| IBIS file generated by GenIBIS.pl Version 3.24
|   j6plus
[IBIS ver]   5.0
[File name]   j6plus.ibs
[File Rev]   1.0.0
[Date]   Thu Jan 25, 2018, 13:15:8
[Source]   Data created at Texas Instruments
[Notes]   J6Plus ABZ IBIS Model Revision History
   Version 1.0.0, January 25th, 2018
   - Initial Release
   Note 1) Checked by IBISCHK5.
[Disclaimer] Please be aware that in the absence of a written agreement,
   Texas Instruments (TI) assumes no liability for: 1) the
   accuracy of the IBIS models provided to your company, 2) the
   proper functioning of these IBIS models in your design or for
   any resulting applications, or, 3) infringement of patents,
   copyrights, or intellectual property rights resulting from
   your use of these IBIS models. TI provides IBIS models as a
   service to our customers and therefore reserves the right to
   limit distribution of the IBIS models.
[Copyright]   Property of Texas Instruments Incorporated. Unauthorised
   reproduction and/or distribution is strictly prohibited. This
   product is protected under copyright law and trade secret law
   as an unpublished work. Created 2016,(C) Copyright 2016,
   Texas Instruments Incorporated., All Rights Reserved. These
   commodities are under the U.S. Government distribution license
   control.As such,they are not to be re-exported without the
   prior approval of the U.S. Department of Commerce.
|   Component j6plus
[Component]   j6plus
[Manufacturer]   Texas Instruments.
| Source IO level model revisions
|Model   Revision   Date
|DDR_SEIOPB_V   2.5   23 May 2014
|BC1833DV40DCPBFBHHVRXP1811_SSCEV   2.0   Sep 11, 2013
|BC1833DV40DCPBFBP1811_SSCEV   2.0   Sep 11, 2013
|BI2C1833DVFZP18_SSCEV   2.0   Sep 11, 2013
|BC1833DV40DCPBFBP1811_SSCEH   2.0   Sep 11, 2013
|DDR_DIFFIOPB_V   2.5   23 May 2014
|SATATX   1.0   Nov 07, 2012
|ACSPCIE_RX   0.5   May 16, 2012
|SDIO1833PB_H   1.0   Sep 21, 2011
|USB3_PCIEGEN1_PCIEGEN2_TX   1.0   Nov 07, 2012
|HDMITXPHY   0.8   Jul 12, 2011
|DDR_DIFFIOPB_H   2.5   23 May 2014
|IQ1833DVTCKPBFBP18LL_SSCEV   2.0   Sep 11, 2013
|BMLBLVDS18_SSCEH   1.0   Jun 13, 2013
|ILVDS18HY_SSCEH   1.0   Apr 04, 2013
|USB2PHYCORE_HMAV10GS80   0.8   July 13, 2011
|GANGARX   1   Sep 04, 2012
|IHHV1833DVHYP1811_SSCEV   1.0   Dec 24, 2012
|DDR_SEIOPB_H   2.5   23 May 2014
[Package]
|   typ   min   max
R_pkg   0.416310963675214   0.029876000000000000 0.885390000000000000
L_pkg   2.57707435897436E-009 0.000000000420200000 0.000000004843000000
C_pkg   1.29004209401709E-012 0.000000000000566900 0.000000000002000000
[Pin]   signal_name   model_name   R_pin   L_pin   C_pin
Y10   ATESTV   NC
G19   DCAN1_RX   Selector_1   0.122460000000000000 0.000000001020000000 0.000000000000844400
G20   DCAN1_TX   Selector_1   0.153960000000000000 0.000000001124000000 0.000000000000940000
Y18   DDR1_VREF0   NC
AC18   DDR1_CASN   Selector_15  0.164920000000000000 0.000000001265000000 0.000000000000943600
AF17   DDR1_BA0   Selector_15  0.301210000000000000 0.000000002001000000 0.000000000001255000
AF24   DDR1_D4   Selector_4   0.467920000000000000 0.000000002978000000 0.000000000001397000
AC27   DDR1_D20   Selector_4   0.577380000000000000 0.000000003559000000 0.000000000001579000
AC24   DDR1_D14   Selector_4   0.366310000000000000 0.000000002279000000 0.000000000001257000
AG25   DDR1_DQSN0   Selector_11  0.686690000000000000 0.000000003636000000 0.000000000001223000
AH25   DDR1_DQS0   Selector_9   0.686670000000000000 0.000000003663000000 0.000000000001216000
AG23   DDR1_A6   Selector_15  0.527210000000000000 0.000000003212000000 0.000000000001560000
AF18   DDR1_A13   Selector_15  0.350510000000000000 0.000000002185000000 0.000000000001282000
AF25   DDR1_D0   Selector_4   0.547110000000000000 0.000000003377000000 0.000000000001490000
Y23   DDR1_D26   Selector_4   0.272260000000000000 0.000000001860000000 0.000000000001192000
AE17   DDR1_A14   Selector_15  0.273350000000000000 0.000000001811000000 0.000000000001053000
AB18   DDR1_BA2   Selector_15  0.110020000000000000 0.000000000951200000 0.000000000000877200
AE28   DDR1_DQSN1   Selector_11  0.760100000000000000 0.000000003994000000 0.000000000001297000
Y22   DDR1_D25   Selector_4   0.243100000000000000 0.000000001796000000 0.000000000001094000
W23   DDR1_ECC_D3   Selector_4   0.310930000000000000 0.000000002177000000 0.000000000001181000
V24   DDR1_ECC_D5   Selector_4   0.304360000000000000 0.000000002061000000 0.000000000001069000
AE23   DDR1_D7   Selector_4   0.349920000000000000 0.000000002264000000 0.000000000001249000
Y26   DDR1_ECC_D7   Selector_4   0.475480000000000000 0.000000002872000000 0.000000000001589000
AF28   DDR1_D11   Selector_4   0.665540000000000000 0.000000003965000000 0.000000000001718000
AF27   DDR1_D9   Selector_4   0.600380000000000000 0.000000003672000000 0.000000000001622000
V25   DDR1_ECC_D6   Selector_4   0.398200000000000000 0.000000002464000000 0.000000000001225000
AB19   DDR1_A3   Selector_15  0.102890000000000000 0.000000000866100000 0.000000000000875200
AB23   DDR1_DQM1   Selector_24  0.300060000000000000 0.000000001913000000 0.000000000001147000
AA26   DDR1_D29   Selector_4   0.444900000000000000 0.000000002759000000 0.000000000001396000
AD21   DDR1_A10   Selector_15  0.232890000000000000 0.000000001597000000 0.000000000001048000
AC20   DDR1_A2   Selector_15  0.179280000000000000 0.000000001323000000 0.000000000001091000
AC19   DDR1_A1   Selector_15  0.195630000000000000 0.000000001384000000 0.000000000001014000
Y19   DDR1_D21   Selector_4   0.124200000000000000 0.000000001407000000 0.000000000000793300
AE21   DDR1_A7   Selector_15  0.276170000000000000 0.000000001894000000 0.000000000001188000
V20   DDR1_D16   Selector_4   0.029876000000000000 0.000000000420200000 0.000000000000566900
W20   DDR1_D17   Selector_4   0.140870000000000000 0.000000001414000000 0.000000000000882900
AC25   DDR1_D13   Selector_4   0.413520000000000000 0.000000002556000000 0.000000000001325000
AF20   DDR1_RASN   Selector_15  0.368020000000000000 0.000000002258000000 0.000000000001267000
AE20   DDR1_ODT0   Selector_15  0.355230000000000000 0.000000002143000000 0.000000000001225000
AC26   DDR1_DQM2   Selector_24  0.480350000000000000 0.000000002974000000 0.000000000001462000
AH21   DDR1_WEN   Selector_15  0.521940000000000000 0.000000003071000000 0.000000000001524000
AF26   DDR1_D1   Selector_4   0.528520000000000000 0.000000003223000000 0.000000000001524000
AA23   DDR1_D24   Selector_4   0.367330000000000000 0.000000002386000000 0.000000000001236000
AE18   DDR1_BA1   Selector_15  0.292490000000000000 0.000000001893000000 0.000000000001142000
AF21   DDR1_A4   Selector_15  0.411750000000000000 0.000000002543000000 0.000000000001330000
Y24   DDR1_D28   Selector_4   0.330980000000000000 0.000000002222000000 0.000000000001202000
AB28   DDR1_D18   Selector_4   0.589030000000000000 0.000000003678000000 0.000000000001605000
AG26   DDR1_D2   Selector_4   0.594910000000000000 0.000000003559000000 0.000000000001617000
AE26   DDR1_D12   Selector_4   0.534150000000000000 0.000000003309000000 0.000000000001512000
W19   DDR1_ECC_D2   Selector_4   0.121200000000000000 0.000000001451000000 0.000000000000911300
Y25   DDR1_ECC_D4   Selector_4   0.438840000000000000 0.000000002766000000 0.000000000001554000
AA24   DDR1_D27   Selector_4   0.365560000000000000 0.000000002344000000 0.000000000001341000
AD25   DDR1_D15   Selector_4   0.440700000000000000 0.000000002662000000 0.000000000001411000
AB27   DDR1_D22   Selector_4   0.526930000000000000 0.000000003352000000 0.000000000001471000
AD18   DDR1_A15   Selector_15  0.256150000000000000 0.000000001762000000 0.000000000001106000
V28   DDR1_DQSN_ECC   Selector_11  0.652950000000000000 0.000000003413000000 0.000000000001116000
AH24   DDR1_NCK   Selector_2   0.675840000000000000 0.000000003620000000 0.000000000001430000
AG21   DDR1_RST   Selector_15  0.485470000000000000 0.000000002873000000 0.000000000001461000
AH26   DDR1_D3   Selector_4   0.636390000000000000 0.000000003722000000 0.000000000001688000
AG27   DDR1_D10   Selector_4   0.660570000000000000 0.000000003855000000 0.000000000001682000
AH23   DDR1_CSN0   Selector_15  0.545150000000000000 0.000000003312000000 0.000000000001572000
V23   DDR1_ECC_D1   Selector_4   0.265250000000000000 0.000000001842000000 0.000000000000989700
AD27   DDR1_DQS2   Selector_9   0.736580000000000000 0.000000003833000000 0.000000000001273000
AD20   DDR1_A0   Selector_15  0.277790000000000000 0.000000001769000000 0.000000000001149000
AE22   DDR1_A9   Selector_15  0.329590000000000000 0.000000002164000000 0.000000000001191000
AC23   DDR1_D8   Selector_4   0.337500000000000000 0.000000002104000000 0.000000000001168000
AF22   DDR1_A8   Selector_15  0.388250000000000000 0.000000002470000000 0.000000000001364000
Y20   DDR1_D23   Selector_4   0.171330000000000000 0.000000001625000000 0.000000000000866800
AA25   DDR1_D30   Selector_4   0.444120000000000000 0.000000002721000000 0.000000000001354000
AE24   DDR1_D5   Selector_4   0.381750000000000000 0.000000002397000000 0.000000000001289000
AA28   DDR1_D31   Selector_4   0.570840000000000000 0.000000003446000000 0.000000000001566000
AD23   DDR1_DQM0   Selector_24  0.413750000000000000 0.000000002529000000 0.000000000001431000
Y28   DDR1_DQS3   Selector_9   0.680200000000000000 0.000000003597000000 0.000000000001212000
AD22   DDR1_A11   Selector_15  0.283590000000000000 0.000000001813000000 0.000000000001127000
W22   DDR1_ECC_D0   Selector_4   0.206760000000000000 0.000000001672000000 0.000000000001080000
AC28   DDR1_D19   Selector_4   0.610720000000000000 0.000000003757000000 0.000000000001645000
V26   DDR1_DQM_ECC   Selector_24  0.391490000000000000 0.000000002463000000 0.000000000001261000
AG24   DDR1_CK   Selector_23  0.669160000000000000 0.000000003598000000 0.000000000001402000
AG22   DDR1_CKE   Selector_15  0.492780000000000000 0.000000002955000000 0.000000000001478000
AE27   DDR1_DQS1   Selector_9   0.755390000000000000 0.000000003951000000 0.000000000001287000
AH22   DDR1_A5   Selector_15  0.522550000000000000 0.000000003169000000 0.000000000001523000
AF23   DDR1_D6   Selector_4   0.435010000000000000 0.000000002668000000 0.000000000001399000
AC21   DDR1_A12   Selector_15  0.134350000000000000 0.000000001044000000 0.000000000000979200
Y27   DDR1_DQSN3   Selector_11  0.684620000000000000 0.000000003563000000 0.000000000001218000
AA27   DDR1_DQM3   Selector_24  0.574580000000000000 0.000000003410000000 0.000000000001518000
AD28   DDR1_DQSN2   Selector_11  0.740220000000000000 0.000000003935000000 0.000000000001267000
V27   DDR1_DQS_ECC   Selector_9   0.648360000000000000 0.000000003393000000 0.000000000001064000
H23   DDR2_D8   Selector_4   0.240810000000000000 0.000000001716000000 0.000000000001047000
G27   DDR2_DQSN0   Selector_11  0.638590000000000000 0.000000003419000000 0.000000000001140000
H24   DDR2_D10   Selector_4   0.233120000000000000 0.000000001629000000 0.000000000000932500
E28   DDR2_D7   Selector_4   0.648570000000000000 0.000000004028000000 0.000000000001696000
T23   DDR2_RASN   Selector_24  0.211170000000000000 0.000000001627000000 0.000000000001110000
T28   DDR2_CK   Selector_19  0.650150000000000000 0.000000003469000000 0.000000000001406000
E26   DDR2_D0   Selector_4   0.521980000000000000 0.000000003242000000 0.000000000001414000
J23   DDR2_D21   Selector_4   0.190720000000000000 0.000000001472000000 0.000000000001064000
P24   DDR2_CSN0   Selector_24  0.246740000000000000 0.000000001653000000 0.000000000001115000
K27   DDR2_DQS2   Selector_9   0.568970000000000000 0.000000003027000000 0.000000000001107000
F24   DDR2_D3   Selector_4   0.244890000000000000 0.000000001861000000 0.000000000001070000
P25   DDR2_A6   Selector_24  0.312340000000000000 0.000000001986000000 0.000000000001205000
L27   DDR2_D24   Selector_4   0.449790000000000000 0.000000002892000000 0.000000000001395000
R24   DDR2_RST   Selector_24  0.241190000000000000 0.000000001815000000 0.000000000000818100
U27   DDR2_BA1   Selector_24  0.486910000000000000 0.000000003017000000 0.000000000001455000
L25   DDR2_D26   Selector_4   0.297020000000000000 0.000000002036000000 0.000000000001162000
H28   DDR2_DQSN1   Selector_11  0.612440000000000000 0.000000003233000000 0.000000000001147000
P22   DDR2_A5   Selector_24  0.108720000000000000 0.000000000951100000 0.000000000000841700
N20   DDR2_A7   Selector_24  0.087295000000000000 0.000000000837800000 0.000000000000973900
U28   DDR2_CASN   Selector_24  0.524570000000000000 0.000000003294000000 0.000000000001509000
R27   DDR2_A3   Selector_24  0.397600000000000000 0.000000002516000000 0.000000000001347000
R28   DDR2_A2   Selector_24  0.476310000000000000 0.000000002942000000 0.000000000001547000
N27   DDR2_A9   Selector_24  0.417770000000000000 0.000000002583000000 0.000000000001359000
J25   DDR2_D13   Selector_4   0.291620000000000000 0.000000001981000000 0.000000000001140000
T27   DDR2_NCK   Selector_6   0.645420000000000000 0.000000003416000000 0.000000000001404000
U22   DDR2_A15   Selector_24  0.216050000000000000 0.000000001636000000 0.000000000000993100
G25   DDR2_D1   Selector_4   0.309710000000000000 0.000000002121000000 0.000000000001364000
N22   DDR2_VREF0   NC
J20   DDR2_D23   Selector_4   0.124920000000000000 0.000000001332000000 0.000000000000792500
P26   DDR2_A11   Selector_24  0.383910000000000000 0.000000002413000000 0.000000000001405000
M26   DDR2_D31   Selector_4   0.362470000000000000 0.000000002349000000 0.000000000001268000
G28   DDR2_DQS0   Selector_9   0.636390000000000000 0.000000003436000000 0.000000000001162000
P27   DDR2_A8   Selector_24  0.441510000000000000 0.000000002655000000 0.000000000001401000
F26   DDR2_D4   Selector_4   0.407610000000000000 0.000000002693000000 0.000000000001340000
J24   DDR2_D15   Selector_4   0.231270000000000000 0.000000001586000000 0.000000000001063000
U26   DDR2_BA2   Selector_24  0.388360000000000000 0.000000002548000000 0.000000000001260000
K20   DDR2_D17   Selector_4   0.110100000000000000 0.000000000960400000 0.000000000000952900
K21   DDR2_D18   Selector_4   0.146240000000000000 0.000000001357000000 0.000000000000769300
F28   DDR2_DQM0   Selector_24  0.485980000000000000 0.000000003089000000 0.000000000001460000
F27   DDR2_D5   Selector_4   0.463800000000000000 0.000000003028000000 0.000000000001403000
H25   DDR2_D9   Selector_4   0.283610000000000000 0.000000001882000000 0.000000000001012000
E27   DDR2_D6   Selector_4   0.697810000000000000 0.000000004197000000 0.000000000001723000
N28   DDR2_A12   Selector_24  0.468070000000000000 0.000000002806000000 0.000000000001458000
M28   DDR2_DQS3   Selector_9   0.612940000000000000 0.000000003288000000 0.000000000001154000
R22   DDR2_A14   Selector_24  0.099049000000000000 0.000000000986200000 0.000000000000850000
F25   DDR2_D2   Selector_4   0.328350000000000000 0.000000002272000000 0.000000000001280000
R23   DDR2_ODT0   Selector_24  0.188980000000000000 0.000000001434000000 0.000000000000996600
U25   DDR2_WEN   Selector_24  0.329990000000000000 0.000000002165000000 0.000000000001199000
P23   DDR2_A4   Selector_24  0.186820000000000000 0.000000001421000000 0.000000000000995300
L22   DDR2_D16   Selector_4   0.160650000000000000 0.000000001265000000 0.000000000000862300
M25   DDR2_D30   Selector_4   0.310970000000000000 0.000000002031000000 0.000000000001158000
K28   DDR2_DQSN2   Selector_11  0.573880000000000000 0.000000003065000000 0.000000000001104000
T22   DDR2_A13   Selector_24  0.131960000000000000 0.000000001064000000 0.000000000000919200
L24   DDR2_D20   Selector_4   0.235900000000000000 0.000000001815000000 0.000000000001064000
U24   DDR2_CKE   Selector_24  0.387060000000000000 0.000000002414000000 0.000000000001258000
G26   DDR2_D12   Selector_4   0.412720000000000000 0.000000002652000000 0.000000000001301000
G24   DDR2_DQM1   Selector_24  0.324140000000000000 0.000000002183000000 0.000000000001192000
M24   DDR2_D29   Selector_4   0.238990000000000000 0.000000001702000000 0.000000000001075000
J26   DDR2_D14   Selector_4   0.365690000000000000 0.000000002376000000 0.000000000001274000
M27   DDR2_DQSN3   Selector_11  0.606620000000000000 0.000000003254000000 0.000000000001143000
L26   DDR2_D25   Selector_4   0.346940000000000000 0.000000002349000000 0.000000000001175000
N23   DDR2_A10   Selector_24  0.166950000000000000 0.000000001245000000 0.000000000001002000
M22   DDR2_DQM3   Selector_24  0.129140000000000000 0.000000001042000000 0.000000000000872100
R26   DDR2_A1   Selector_24  0.438110000000000000 0.000000002781000000 0.000000000001390000
H27   DDR2_DQS1   Selector_9   0.606290000000000000 0.000000003215000000 0.000000000001140000
H26   DDR2_D11   Selector_4   0.376180000000000000 0.000000002442000000 0.000000000001044000
K22   DDR2_D22   Selector_4   0.151900000000000000 0.000000001300000000 0.000000000000851000
M23   DDR2_D28   Selector_4   0.191100000000000000 0.000000001538000000 0.000000000000994800
R25   DDR2_A0   Selector_24  0.295990000000000000 0.000000001946000000 0.000000000001164000
K23   DDR2_DQM2   Selector_24  0.193660000000000000 0.000000001440000000 0.000000000000942300
L23   DDR2_D19   Selector_4   0.160130000000000000 0.000000001405000000 0.000000000000860500
U23   DDR2_BA0   Selector_24  0.217440000000000000 0.000000001679000000 0.000000000001004000
L28   DDR2_D27   Selector_4   0.467880000000000000 0.000000003012000000 0.000000000001388000
G21   EMU0   Selector_1   0.210670000000000000 0.000000001513000000 0.000000000001052000
D24   EMU1   Selector_1   0.610690000000000000 0.000000003477000000 0.000000000001687000
F20   GPIO6_15   Selector_1   0.217870000000000000 0.000000001581000000 0.000000000001032000
AB4   GPIO6_11   Selector_3   0.453040000000000000 0.000000002776000000 0.000000000001450000
E21   GPIO6_14   Selector_1   0.299290000000000000 0.000000001976000000 0.000000000001117000
AC5   GPIO6_10   Selector_3   0.515360000000000000 0.000000003043000000 0.000000000001473000
F21   GPIO6_16   Selector_1   0.266490000000000000 0.000000001815000000 0.000000000001092000
J4   GPMC_A24   Selector_3   0.291730000000000000 0.000000001896000000 0.000000000001168000
P1   GPMC_CS3   Selector_3   0.528930000000000000 0.000000003226000000 0.000000000001523000
M1   GPMC_AD3   Selector_3   0.477430000000000000 0.000000002985000000 0.000000000001442000
T2   GPMC_A14   Selector_3   0.492150000000000000 0.000000002952000000 0.000000000001463000
M7   GPMC_A20   Selector_3   0.156510000000000000 0.000000001381000000 0.000000000000860800
H2   GPMC_AD14   Selector_3   0.470220000000000000 0.000000002899000000 0.000000000001439000
J3   GPMC_AD13   Selector_3   0.360410000000000000 0.000000002239000000 0.000000000001258000
J1   GPMC_AD10   Selector_3   0.492680000000000000 0.000000002999000000 0.000000000001450000
J7   GPMC_A23   Selector_3   0.098787000000000000 0.000000000927100000 0.000000000000827700
P7   GPMC_CLK   Selector_3   0.121860000000000000 0.000000001057000000 0.000000000001006000
N6   GPMC_BEN0   Selector_3   0.206180000000000000 0.000000001474000000 0.000000000001071000
T6   GPMC_A2   Selector_3   0.308980000000000000 0.000000002202000000 0.000000000001105000
H5   GPMC_A27   Selector_3   0.251850000000000000 0.000000001711000000 0.000000000001110000
T1   GPMC_CS0   Selector_3   0.599210000000000000 0.000000003538000000 0.000000000001612000
T9   GPMC_A1   Selector_3   0.343020000000000000 0.000000002821000000 0.000000000001436000
M4   GPMC_BEN1   Selector_3   0.300700000000000000 0.000000001986000000 0.000000000001158000
H4   GPMC_A26   Selector_3   0.296060000000000000 0.000000001958000000 0.000000000001176000
L1   GPMC_AD8   Selector_3   0.492080000000000000 0.000000003001000000 0.000000000001454000
R9   GPMC_A5   Selector_3   0.197610000000000000 0.000000001861000000 0.000000000000991500
J5   GPMC_A21   Selector_3   0.237000000000000000 0.000000001696000000 0.000000000001036000
M3   GPMC_WEN   Selector_3   0.371310000000000000 0.000000002441000000 0.000000000001276000
K7   GPMC_A19   Selector_3   0.111770000000000000 0.000000001116000000 0.000000000000855500
P3   GPMC_A17   Selector_3   0.402580000000000000 0.000000002572000000 0.000000000001333000
K2   GPMC_AD9   Selector_3   0.395330000000000000 0.000000002415000000 0.000000000001328000
L5   GPMC_AD2   Selector_3   0.263700000000000000 0.000000001806000000 0.000000000001092000
R4   GPMC_A9   Selector_3   0.384180000000000000 0.000000002422000000 0.000000000001310000
H3   GPMC_AD15   Selector_3   0.403470000000000000 0.000000002535000000 0.000000000001326000
M5   GPMC_OEN_REN   Selector_3   0.234930000000000000 0.000000001637000000 0.000000000001073000
M6   GPMC_AD0   Selector_3   0.260090000000000000 0.000000001821000000 0.000000000001146000
R6   GPMC_A0   Selector_3   0.288940000000000000 0.000000001989000000 0.000000000001085000
M2   GPMC_AD1   Selector_3   0.412900000000000000 0.000000002609000000 0.000000000001347000
T7   GPMC_A3   Selector_3   0.241280000000000000 0.000000001799000000 0.000000000001191000
N2   GPMC_WAIT0   Selector_3   0.427140000000000000 0.000000002701000000 0.000000000001366000
P6   GPMC_A4   Selector_3   0.194950000000000000 0.000000001458000000 0.000000000000890200
K6   GPMC_A22   Selector_3   0.205000000000000000 0.000000001568000000 0.000000000001025000
R5   GPMC_A6   Selector_3   0.339370000000000000 0.000000002271000000 0.000000000001307000
L4   GPMC_AD5   Selector_3   0.275690000000000000 0.000000001812000000 0.000000000001154000
P2   GPMC_CS2   Selector_3   0.439120000000000000 0.000000002752000000 0.000000000001408000
J2   GPMC_AD11   Selector_3   0.412050000000000000 0.000000002557000000 0.000000000001335000
L6   GPMC_AD4   Selector_3   0.268580000000000000 0.000000001799000000 0.000000000001168000
N1   GPMC_ADVN_ALE   Selector_3   0.517060000000000000 0.000000003232000000 0.000000000001496000
P5   GPMC_A7   Selector_3   0.276060000000000000 0.000000001849000000 0.000000000000872300
J6   GPMC_A25   Selector_3   0.191900000000000000 0.000000001431000000 0.000000000000966200
L2   GPMC_AD7   Selector_3   0.401480000000000000 0.000000002515000000 0.000000000001340000
L3   GPMC_AD6   Selector_3   0.358640000000000000 0.000000002324000000 0.000000000001271000
H6   GPMC_CS1   Selector_3   0.168370000000000000 0.000000001280000000 0.000000000000964700
R3   GPMC_A13   Selector_3   0.426150000000000000 0.000000002676000000 0.000000000001378000
U2   GPMC_A15   Selector_3   0.577050000000000000 0.000000003437000000 0.000000000001609000
U1   GPMC_A16   Selector_3   0.588670000000000000 0.000000003468000000 0.000000000001629000
N9   GPMC_A10   Selector_3   0.167700000000000000 0.000000001421000000 0.000000000000893300
R2   GPMC_A18   Selector_3   0.477360000000000000 0.000000002858000000 0.000000000001460000
P4   GPMC_A12   Selector_3   0.317910000000000000 0.000000002057000000 0.000000000001226000
N7   GPMC_A8   Selector_3   0.176810000000000000 0.000000001368000000 0.000000000000797400
P9   GPMC_A11   Selector_3   0.154040000000000000 0.000000001316000000 0.000000000000863000
H1   GPMC_AD12   Selector_3   0.619770000000000000 0.000000003715000000 0.000000000001581000
AH16   HDMI1_CLOCKY   ibis_tmdsm_M#44   0.571920000000000000 0.000000003071000000 0.000000000001110000
AH19   HDMI1_DATA2Y   ibis_tmdsm_M#44   0.649690000000000000 0.000000003339000000 0.000000000001189000
AH17   HDMI1_DATA0Y   ibis_tmdsm_M#44   0.568420000000000000 0.000000003074000000 0.000000000001104000
AH18   HDMI1_DATA1Y   ibis_tmdsm_M#44   0.613430000000000000 0.000000003241000000 0.000000000001156000
AG18   HDMI1_DATA1X   ibis_tmdsp_M#43   0.607690000000000000 0.000000003192000000 0.000000000001158000
AG17   HDMI1_DATA0X   ibis_tmdsp_M#43   0.557830000000000000 0.000000003023000000 0.000000000001077000
AG16   HDMI1_CLOCKX   ibis_tmdsp_M#43   0.561720000000000000 0.000000003002000000 0.000000000001066000
AG19   HDMI1_DATA2X   ibis_tmdsp_M#43   0.646780000000000000 0.000000003295000000 0.000000000001187000
C20   I2C1_SCL   Selector_21  0.392320000000000000 0.000000002451000000 0.000000000001342000
C25   I2C2_SDA   Selector_21  0.683350000000000000 0.000000003941000000 0.000000000001770000
F17   I2C2_SCL   Selector_21  0.175220000000000000 0.000000001289000000 0.000000000001037000
C21   I2C1_SDA   Selector_21  0.429010000000000000 0.000000002605000000 0.000000000001399000
AG15   LJCB_CLKP   ACSPCIE_RX_M#753   0.558230000000000000 0.000000003040000000 0.000000000001286000
AH15   LJCB_CLKN   ACSPCIE_RX_M#753   0.576810000000000000 0.000000003218000000 0.000000000001301000
F14   MCASP1_AXR15   Selector_1   0.190290000000000000 0.000000001469000000 0.000000000000967800
J14   MCASP1_FSR   Selector_1   0.086283000000000000 0.000000000988700000 0.000000000000881600
A12   MCASP1_AXR11   Selector_1   0.509860000000000000 0.000000003239000000 0.000000000001463000
G12   MCASP1_AXR0   Selector_1   0.096733000000000000 0.000000000857600000 0.000000000000847800
B12   MCASP1_AXR8   Selector_1   0.402560000000000000 0.000000002602000000 0.000000000001334000
A11   MCASP1_AXR9   Selector_1   0.518700000000000000 0.000000003316000000 0.000000000001489000
C12   MCASP1_AXR6   Selector_1   0.355690000000000000 0.000000002295000000 0.000000000001244000
G13   MCASP1_AXR2   Selector_1   0.076957000000000000 0.000000000819900000 0.000000000000812800
A13   MCASP1_AXR13   Selector_1   0.480130000000000000 0.000000003007000000 0.000000000001427000
G14   MCASP1_AXR14   Selector_1   0.077843000000000000 0.000000000814500000 0.000000000000771000
F13   MCASP1_AXR5   Selector_1   0.170500000000000000 0.000000001298000000 0.000000000000921700
C14   MCASP1_ACLKX   Selector_1   0.346490000000000000 0.000000002246000000 0.000000000001229000
D12   MCASP1_AXR7   Selector_1   0.320340000000000000 0.000000002092000000 0.000000000001152000
B13   MCASP1_AXR10   Selector_1   0.386000000000000000 0.000000002502000000 0.000000000001276000
E14   MCASP1_AXR12   Selector_1   0.218290000000000000 0.000000001518000000 0.000000000001036000
F12   MCASP1_AXR1   Selector_1   0.186440000000000000 0.000000001508000000 0.000000000000984500
E12   MCASP1_AXR4   Selector_1   0.219410000000000000 0.000000001479000000 0.000000000001057000
D14   MCASP1_FSX   Selector_1   0.260650000000000000 0.000000001753000000 0.000000000001137000
J11   MCASP1_AXR3   Selector_1   0.150440000000000000 0.000000001402000000 0.000000000001091000
B14   MCASP1_ACLKR   Selector_1   0.380010000000000000 0.000000002357000000 0.000000000001292000
A20   MCASP2_FSR   Selector_1   0.708330000000000000 0.000000004296000000 0.000000000001766000
E15   MCASP2_ACLKR   Selector_1   0.201150000000000000 0.000000001406000000 0.000000000001029000
C15   MCASP2_AXR2   Selector_1   0.342120000000000000 0.000000002164000000 0.000000000001222000
A19   MCASP2_ACLKX   Selector_1   0.566880000000000000 0.000000003498000000 0.000000000001593000
A17   MCASP2_AXR7   Selector_1   0.553650000000000000 0.000000003422000000 0.000000000001572000
B15   MCASP2_AXR0   Selector_1   0.385200000000000000 0.000000002385000000 0.000000000001313000
B17   MCASP2_AXR6   Selector_1   0.470300000000000000 0.000000002989000000 0.000000000001432000
B16   MCASP2_AXR5   Selector_1   0.458270000000000000 0.000000002833000000 0.000000000001400000
A16   MCASP2_AXR3   Selector_1   0.507840000000000000 0.000000003115000000 0.000000000001494000
D15   MCASP2_AXR4   Selector_1   0.281870000000000000 0.000000001718000000 0.000000000001139000
A18   MCASP2_FSX   Selector_1   0.589690000000000000 0.000000003622000000 0.000000000001596000
A15   MCASP2_AXR1   Selector_1   0.479020000000000000 0.000000002865000000 0.000000000001472000
C17   MCASP3_AXR1   Selector_1   0.359750000000000000 0.000000002305000000 0.000000000001310000
F15   MCASP3_FSX   Selector_1   0.210910000000000000 0.000000001494000000 0.000000000001057000
B18   MCASP3_ACLKX   Selector_1   0.457210000000000000 0.000000002865000000 0.000000000001458000
B19   MCASP3_AXR0   Selector_1   0.514140000000000000 0.000000003138000000 0.000000000001497000
A21   MCASP4_FSX   Selector_1   0.611460000000000000 0.000000003634000000 0.000000000001675000
C18   MCASP4_ACLKX   Selector_1   0.493680000000000000 0.000000002970000000 0.000000000001441000
D17   MCASP4_AXR1   Selector_1   0.325750000000000000 0.000000002066000000 0.000000000001225000
G16   MCASP4_AXR0   Selector_1   0.076727000000000000 0.000000000726000000 0.000000000000842000
AB9   MCASP5_FSX   Selector_3   0.427290000000000000 0.000000003018000000 0.000000000001279000
AB3   MCASP5_AXR0   Selector_3   0.525870000000000000 0.000000003124000000 0.000000000001554000
AA3   MCASP5_ACLKX   Selector_3   0.470920000000000000 0.000000002967000000 0.000000000001422000
AA4   MCASP5_AXR1   Selector_3   0.414350000000000000 0.000000002573000000 0.000000000001374000
V1   MDIO_MCLK   Selector_3   0.575280000000000000 0.000000003382000000 0.000000000001595000
U4   MDIO_D   Selector_3   0.363390000000000000 0.000000002348000000 0.000000000001358000
AA1   MLBP_DAT_P   Selector_8   0.781090000000000000 0.000000004160000000 0.000000000001226000
AC1   MLBP_SIG_P   Selector_8   0.885390000000000000 0.000000004408000000 0.000000000001421000
AB2   MLBP_CLK_N   Selector_17  0.835580000000000000 0.000000004318000000 0.000000000001591000
AC2   MLBP_SIG_N   Selector_8   0.879920000000000000 0.000000004425000000 0.000000000001432000
AB1   MLBP_CLK_P   Selector_17  0.842990000000000000 0.000000004299000000 0.000000000001596000
AA2   MLBP_DAT_N   Selector_8   0.773220000000000000 0.000000004134000000 0.000000000001228000
Y9   MMC1_SDWP   Selector_3   0.191560000000000000 0.000000001936000000 0.000000000001015000
AA5   MMC1_DAT2   Selector_10  0.420790000000000000 0.000000002707000000 0.000000000001413000
W7   MMC1_SDCD   Selector_3   0.246510000000000000 0.000000001530000000 0.000000000000995200
W6   MMC1_CLK   Selector_10  0.283310000000000000 0.000000001911000000 0.000000000001270000
Y3   MMC1_DAT3   Selector_10  0.451260000000000000 0.000000002587000000 0.000000000001476000
Y4   MMC1_DAT1   Selector_10  0.378740000000000000 0.000000002378000000 0.000000000001391000
Y6   MMC1_CMD   Selector_10  0.355210000000000000 0.000000002326000000 0.000000000001405000
AA6   MMC1_DAT0   Selector_10  0.445360000000000000 0.000000002962000000 0.000000000001431000
AC6   MMC3_DAT1   Selector_3   0.462550000000000000 0.000000002769000000 0.000000000001117000
AC8   MMC3_DAT4   Selector_3   0.501240000000000000 0.000000003198000000 0.000000000001483000
AC3   MMC3_DAT3   Selector_3   0.559820000000000000 0.000000003309000000 0.000000000001605000
AB5   MMC3_DAT7   Selector_3   0.399900000000000000 0.000000002478000000 0.000000000001330000
AC7   MMC3_DAT0   Selector_3   0.405150000000000000 0.000000002579000000 0.000000000001270000
AD6   MMC3_DAT5   Selector_3   0.499280000000000000 0.000000002984000000 0.000000000001556000
AC4   MMC3_CMD   Selector_3   0.528400000000000000 0.000000003167000000 0.000000000001530000
AC9   MMC3_DAT2   Selector_3   0.471100000000000000 0.000000003188000000 0.000000000001446000
AB8   MMC3_DAT6   Selector_3   0.396960000000000000 0.000000002795000000 0.000000000001086000
AD4   MMC3_CLK   Selector_3   0.538290000000000000 0.000000003176000000 0.000000000001549000
D21   NMIN   Selector_20  0.365900000000000000 0.000000002288000000 0.000000000001287000
Y11   ON_OFF   Selector_16  0.179250000000000000 0.000000001754000000 0.000000000000818900
AG13   PCIE_RXN0   usb3rx_M#227   0.531380000000000000 0.000000002953000000 0.000000000001044000
AG14   PCIE_TXN0   Selector_22  0.556410000000000000 0.000000003016000000 0.000000000001102000
AG12   PCIE_TXN1   Selector_22  0.518000000000000000 0.000000002903000000 0.000000000001015000
AH12   PCIE_TXP1   Selector_7   0.530450000000000000 0.000000002963000000 0.000000000001058000
AH14   PCIE_TXP0   Selector_7   0.569920000000000000 0.000000003126000000 0.000000000001098000
AG11   PCIE_RXN1   usb3rx_M#227   0.558570000000000000 0.000000003010000000 0.000000000001092000
AH13   PCIE_RXP0   usb3rx_M#227   0.542350000000000000 0.000000003012000000 0.000000000001069000
AH11   PCIE_RXP1   usb3rx_M#227   0.563190000000000000 0.000000003075000000 0.000000000001090000
F22   PORZ   Selector_14  0.354010000000000000 0.000000002167000000 0.000000000001286000
E23   RESETN   Selector_20  0.460550000000000000 0.000000002729000000 0.000000000001422000
W9   RGMII0_TXC   Selector_3   0.258630000000000000 0.000000002697000000 0.000000000001209000
V3   RGMII0_RXD2   Selector_3   0.458120000000000000 0.000000002759000000 0.000000000001455000
V6   RGMII0_TXD1   Selector_3   0.283890000000000000 0.000000002098000000 0.000000000001213000
V4   RGMII0_RXD3   Selector_3   0.367210000000000000 0.000000002569000000 0.000000000001400000
U5   RGMII0_RXC   Selector_3   0.301060000000000000 0.000000002086000000 0.000000000001273000
V5   RGMII0_RXCTL   Selector_3   0.306540000000000000 0.000000002144000000 0.000000000001199000
U7   RGMII0_TXD2   Selector_3   0.183830000000000000 0.000000001727000000 0.000000000000992500
U6   RGMII0_TXD0   Selector_3   0.255220000000000000 0.000000001952000000 0.000000000001044000
V9   RGMII0_TXCTL   Selector_3   0.211760000000000000 0.000000002050000000 0.000000000001075000
V7   RGMII0_TXD3   Selector_3   0.265520000000000000 0.000000002023000000 0.000000000001220000
W2   RGMII0_RXD0   Selector_3   0.565410000000000000 0.000000003231000000 0.000000000001613000
Y2   RGMII0_RXD1   Selector_3   0.604960000000000000 0.000000003536000000 0.000000000001663000
U3   RMII_MHZ_50_CLK   Selector_3   0.436800000000000000 0.000000002686000000 0.000000000001388000
F23   RSTOUTN   Selector_5   0.441700000000000000 0.000000002586000000 0.000000000001410000
AD14   RTC_OSC_XO   NC
AF14   RTC_ISO   Selector_14  0.336170000000000000 0.000000002277000000 0.000000000001204000
AB17   RTC_PORZ   Selector_14  0.129750000000000000 0.000000001225000000 0.000000000000787600
AE14   RTC_OSC_XI_CLKIN32   NC
E18   RTCK   Selector_5   0.224230000000000000 0.000000001557000000 0.000000000001079000
AG9   SATA1_RXP0   usb3rx_M#227   0.604150000000000000 0.000000003183000000 0.000000000001105000
AH10   SATA1_TXP0   sata_tx_M#752   0.576430000000000000 0.000000003093000000 0.000000000001105000
AH9   SATA1_RXN0   usb3rx_M#227   0.605090000000000000 0.000000003165000000 0.000000000001136000
AG10   SATA1_TXN0   sata_tx_M#752   0.567160000000000000 0.000000003086000000 0.000000000001069000
B20   SPI1_CS3   Selector_1   0.496050000000000000 0.000000002978000000 0.000000000001515000
A25   SPI1_SCLK   Selector_1   0.787960000000000000 0.000000004556000000 0.000000000001948000
F16   SPI1_D1   Selector_1   0.142940000000000000 0.000000001120000000 0.000000000000989800
A24   SPI1_CS0   Selector_1   0.769980000000000000 0.000000004267000000 0.000000000001919000
B21   SPI1_CS2   Selector_1   0.528490000000000000 0.000000003101000000 0.000000000001554000
A22   SPI1_CS1   Selector_1   0.652610000000000000 0.000000003696000000 0.000000000001733000
B25   SPI1_D0   Selector_1   0.810960000000000000 0.000000004560000000 0.000000000001990000
A26   SPI2_SCLK   Selector_1   0.849820000000000000 0.000000004843000000 0.000000000001993000
B22   SPI2_D1   Selector_1   0.584400000000000000 0.000000003383000000 0.000000000001634000
B24   SPI2_CS0   Selector_1   0.701580000000000000 0.000000003903000000 0.000000000001840000
G17   SPI2_D0   Selector_1   0.056831000000000000 0.000000000712400000 0.000000000000827500
E20   TCLK   Selector_12  0.295540000000000000 0.000000001906000000 0.000000000001138000
D23   TDI   Selector_20  0.527150000000000000 0.000000003065000000 0.000000000001540000
F19   TDO   Selector_5   0.196280000000000000 0.000000001345000000 0.000000000000994000
F18   TMS   Selector_20  0.190300000000000000 0.000000001326000000 0.000000000000976600
D20   TRSTN   Selector_20  0.322270000000000000 0.000000001987000000 0.000000000001184000
B27   UART1_RXD   Selector_1   0.686360000000000000 0.000000003917000000 0.000000000001721000
E25   UART1_CTSN   Selector_1   0.486850000000000000 0.000000002961000000 0.000000000001425000
C27   UART1_RTSN   Selector_1   0.651470000000000000 0.000000003794000000 0.000000000001703000
C26   UART1_TXD   Selector_1   0.608100000000000000 0.000000003623000000 0.000000000001603000
D27   UART2_CTSN   Selector_1   0.592850000000000000 0.000000003685000000 0.000000000001582000
D28   UART2_RXD   Selector_1   0.656850000000000000 0.000000004017000000 0.000000000001678000
D26   UART2_TXD   Selector_1   0.551860000000000000 0.000000003356000000 0.000000000001546000
C28   UART2_RTSN   Selector_1   0.703820000000000000 0.000000004178000000 0.000000000001726000
Y1   UART3_TXD   Selector_3   0.654740000000000000 0.000000003698000000 0.000000000001703000
V2   UART3_RXD   Selector_3   0.531070000000000000 0.000000003145000000 0.000000000001531000
AF12   USB_RXN0   usb3rx_M#227   0.355930000000000000 0.000000002364000000 0.000000000001064000
AD11   USB_TXP0   Selector_7   0.262330000000000000 0.000000001701000000 0.000000000000872400
AE12   USB_RXP0   usb3rx_M#227   0.348500000000000000 0.000000002272000000 0.000000000001044000
AC11   USB_TXN0   Selector_22  0.264110000000000000 0.000000001718000000 0.000000000000859300
AB10   USB1_DRVVBUS   Selector_3   0.222820000000000000 0.000000001650000000 0.000000000000936900
AD12   USB1_DP   Selector_13  0.245510000000000000 0.000000001902000000 0.000000000001012000
AC12   USB1_DM   Selector_18  0.230880000000000000 0.000000001907000000 0.000000000001013000
AE11   USB2_DP   Selector_13  0.406130000000000000 0.000000002386000000 0.000000000001033000
AF11   USB2_DM   Selector_18  0.414690000000000000 0.000000002457000000 0.000000000001031000
AC10   USB2_DRVVBUS   Selector_3   0.232040000000000000 0.000000001753000000 0.000000000000961100
AG4   VIN1A_D8   Selector_3   0.644140000000000000 0.000000003768000000 0.000000000001745000
AG8   VIN1A_CLK0   Selector_3   0.456950000000000000 0.000000002811000000 0.000000000001382000
AE2   VIN1A_D20   Selector_3   0.705280000000000000 0.000000004135000000 0.000000000001794000
AE9   VIN1A_HSYNC0   Selector_3   0.343420000000000000 0.000000002201000000 0.000000000001284000
AF3   VIN1A_D14   Selector_3   0.709310000000000000 0.000000004142000000 0.000000000001772000
AG5   VIN1A_D11   Selector_3   0.612550000000000000 0.000000003636000000 0.000000000001668000
AE5   VIN1A_D18   Selector_3   0.541150000000000000 0.000000003229000000 0.000000000001581000
AH3   VIN1A_D4   Selector_3   0.723470000000000000 0.000000004088000000 0.000000000001860000
AH7   VIN1B_CLK1   Selector_3   0.518630000000000000 0.000000003116000000 0.000000000001473000
AG3   VIN1A_D10   Selector_3   0.722080000000000000 0.000000004143000000 0.000000000001848000
AF6   VIN1A_D13   Selector_3   0.557040000000000000 0.000000003335000000 0.000000000001558000
AF2   VIN1A_D12   Selector_3   0.739150000000000000 0.000000004170000000 0.000000000001899000
AE3   VIN1A_D17   Selector_3   0.610430000000000000 0.000000003619000000 0.000000000001679000
AG6   VIN1A_D6   Selector_3   0.560780000000000000 0.000000003377000000 0.000000000001594000
AH4   VIN1A_D7   Selector_3   0.685090000000000000 0.000000004037000000 0.000000000001791000
AF8   VIN1A_VSYNC0   Selector_3   0.433520000000000000 0.000000002615000000 0.000000000001417000
AF4   VIN1A_D15   Selector_3   0.614510000000000000 0.000000003576000000 0.000000000001665000
AE1   VIN1A_D19   Selector_3   0.733440000000000000 0.000000004273000000 0.000000000001879000
AE6   VIN1A_D21   Selector_3   0.511380000000000000 0.000000003177000000 0.000000000001483000
AD3   VIN1A_D23   Selector_3   0.623830000000000000 0.000000003860000000 0.000000000001639000
AD8   VIN1A_D1   Selector_3   0.290910000000000000 0.000000001865000000 0.000000000001133000
AF1   VIN1A_D16   Selector_3   0.818720000000000000 0.000000004565000000 0.000000000002000000
AG7   VIN1A_D2   Selector_3   0.501510000000000000 0.000000002956000000 0.000000000001484000
AF9   VIN1A_FLD0   Selector_3   0.425880000000000000 0.000000002833000000 0.000000000001425000
AG2   VIN1A_D9   Selector_3   0.762120000000000000 0.000000004188000000 0.000000000001921000
AH5   VIN1A_D5   Selector_3   0.623950000000000000 0.000000003706000000 0.000000000001726000
AH6   VIN1A_D3   Selector_3   0.600380000000000000 0.000000003620000000 0.000000000001657000
AE8   VIN1A_D0   Selector_3   0.390070000000000000 0.000000002410000000 0.000000000001280000
AD2   VIN1A_D22   Selector_3   0.654400000000000000 0.000000003917000000 0.000000000001660000
AD9   VIN1A_DE0   Selector_3   0.268050000000000000 0.000000001969000000 0.000000000001134000
C4   VIN2A_D15   Selector_1   0.511230000000000000 0.000000003069000000 0.000000000001533000
C5   VIN2A_D18   Selector_1   0.480720000000000000 0.000000002882000000 0.000000000001486000
B3   VIN2A_D20   Selector_1   0.642120000000000000 0.000000003706000000 0.000000000001600000
F6   VIN2A_D11   Selector_1   0.316620000000000000 0.000000002010000000 0.000000000001196000
F3   VIN2A_D1   Selector_1   0.444350000000000000 0.000000002731000000 0.000000000001385000
E4   VIN2A_D7   Selector_1   0.418800000000000000 0.000000002532000000 0.000000000001369000
B2   VIN2A_D16   Selector_1   0.673200000000000000 0.000000003755000000 0.000000000001756000
A4   VIN2A_D23   Selector_1   0.631730000000000000 0.000000003677000000 0.000000000001681000
E1   VIN2A_CLK0   Selector_1   0.551850000000000000 0.000000003191000000 0.000000000001568000
D3   VIN2A_D10   Selector_1   0.531630000000000000 0.000000003156000000 0.000000000001548000
C3   VIN2A_D14   Selector_1   0.553320000000000000 0.000000003274000000 0.000000000001586000
D2   VIN2A_D4   Selector_1   0.546620000000000000 0.000000003238000000 0.000000000001578000
C1   VIN2A_D6   Selector_1   0.660820000000000000 0.000000003779000000 0.000000000001730000
G2   VIN2A_DE0   Selector_1   0.440660000000000000 0.000000002654000000 0.000000000001401000
F2   VIN2A_D0   Selector_1   0.481100000000000000 0.000000002842000000 0.000000000001430000
E6   VIN2A_D9   Selector_1   0.319700000000000000 0.000000001995000000 0.000000000001193000
C2   VIN2A_D13   Selector_1   0.612930000000000000 0.000000003553000000 0.000000000001570000
B4   VIN2A_D21   Selector_1   0.594510000000000000 0.000000003528000000 0.000000000001637000
E2   VIN2A_D3   Selector_1   0.521090000000000000 0.000000003053000000 0.000000000001528000
A3   VIN2A_D19   Selector_1   0.706960000000000000 0.000000003981000000 0.000000000001836000
D6   VIN2A_D17   Selector_1   0.378640000000000000 0.000000002353000000 0.000000000001312000
D1   VIN2A_D2   Selector_1   0.594670000000000000 0.000000003478000000 0.000000000001643000
D5   VIN2A_D12   Selector_1   0.399700000000000000 0.000000002471000000 0.000000000001323000
F5   VIN2A_D8   Selector_1   0.343010000000000000 0.000000002144000000 0.000000000001260000
B5   VIN2A_D22   Selector_1   0.526690000000000000 0.000000003082000000 0.000000000001533000
G6   VIN2A_VSYNC0   Selector_1   0.209530000000000000 0.000000001429000000 0.000000000001050000
G1   VIN2A_HSYNC0   Selector_1   0.493400000000000000 0.000000002895000000 0.000000000001474000
H7   VIN2A_FLD0   Selector_1   0.106300000000000000 0.000000000881100000 0.000000000000856300
F4   VIN2A_D5   Selector_1   0.391250000000000000 0.000000002425000000 0.000000000001329000
A8   VOUT1_D19   Selector_1   0.530670000000000000 0.000000003221000000 0.000000000001549000
E7   VOUT1_D7   Selector_1   0.383540000000000000 0.000000002382000000 0.000000000001351000
B8   VOUT1_D17   Selector_1   0.463940000000000000 0.000000002853000000 0.000000000001450000
B11   VOUT1_FLD   Selector_1   0.419930000000000000 0.000000002678000000 0.000000000001364000
C9   VOUT1_D20   Selector_1   0.415950000000000000 0.000000002694000000 0.000000000001327000
D9   VOUT1_D9   Selector_1   0.314710000000000000 0.000000002033000000 0.000000000001184000
C6   VOUT1_D13   Selector_1   0.538220000000000000 0.000000003168000000 0.000000000001528000
F10   VOUT1_D2   Selector_1   0.148300000000000000 0.000000001140000000 0.000000000000954900
F8   VOUT1_D6   Selector_1   0.362190000000000000 0.000000002239000000 0.000000000001301000
G11   VOUT1_D3   Selector_1   0.102570000000000000 0.000000000940500000 0.000000000000854500
B10   VOUT1_DE   Selector_1   0.457370000000000000 0.000000002943000000 0.000000000001364000
A5   VOUT1_D12   Selector_1   0.661750000000000000 0.000000003757000000 0.000000000001739000
F9   VOUT1_D5   Selector_1   0.307330000000000000 0.000000001950000000 0.000000000001215000
A9   VOUT1_D21   Selector_1   0.512710000000000000 0.000000003171000000 0.000000000001506000
E11   VOUT1_VSYNC   Selector_1   0.276370000000000000 0.000000001878000000 0.000000000001135000
B9   VOUT1_D22   Selector_1   0.470440000000000000 0.000000003015000000 0.000000000001393000
E8   VOUT1_D8   Selector_1   0.353540000000000000 0.000000002239000000 0.000000000001273000
E9   VOUT1_D4   Selector_1   0.254110000000000000 0.000000001732000000 0.000000000001108000
D7   VOUT1_D10   Selector_1   0.454260000000000000 0.000000002778000000 0.000000000001428000
C11   VOUT1_HSYNC   Selector_1   0.389250000000000000 0.000000002573000000 0.000000000001265000
A7   VOUT1_D18   Selector_1   0.575250000000000000 0.000000003342000000 0.000000000001617000
C7   VOUT1_D15   Selector_1   0.497340000000000000 0.000000002985000000 0.000000000001513000
F11   VOUT1_D0   Selector_1   0.115820000000000000 0.000000001074000000 0.000000000000945700
A10   VOUT1_D23   Selector_1   0.494740000000000000 0.000000003097000000 0.000000000001475000
C8   VOUT1_D14   Selector_1   0.413390000000000000 0.000000002614000000 0.000000000001344000
D11   VOUT1_CLK   Selector_1   0.286790000000000000 0.000000001886000000 0.000000000001159000
G10   VOUT1_D1   Selector_1   0.115200000000000000 0.000000001071000000 0.000000000000879500
B7   VOUT1_D16   Selector_1   0.538400000000000000 0.000000003178000000 0.000000000001538000
D8   VOUT1_D11   Selector_1   0.412730000000000000 0.000000002586000000 0.000000000001344000
AD17   WAKEUP0   Selector_14  0.238090000000000000 0.000000001827000000 0.000000000001072000
AC17   WAKEUP1   Selector_14  0.191410000000000000 0.000000001631000000 0.000000000000973300
AB16   WAKEUP2   Selector_14  0.144160000000000000 0.000000001263000000 0.000000000000744800
AC16   WAKEUP3   Selector_14  0.201280000000000000 0.000000001613000000 0.000000000000954500
AC15   XI_OSC1   NC
AE15   XI_OSC0   NC
AD15   XO_OSC0   NC
AC13   XO_OSC1   NC
B26   XREF_CLK2   Selector_1   0.779580000000000000 0.000000004521000000 0.000000000001918000
D18   XREF_CLK0   Selector_1   0.345230000000000000 0.000000002114000000 0.000000000001279000
C23   XREF_CLK3   Selector_1   0.602840000000000000 0.000000003553000000 0.000000000001623000
E17   XREF_CLK1   Selector_1   0.264110000000000000 0.000000001752000000 0.000000000001123000
[Diff Pin] inv_pin vdiff tdelay_typ tdelay_min tdelay_max
|Differential signal data for cell USB3_PCIEGEN1_PCIEGEN2_TX
|PCIE_TXP1   PCIE_TXN1
AH12   AG12   200m   0
|USB_TXP0   USB_TXN0
AD11   AC11   200m   0
|PCIE_TXP0   PCIE_TXN0
AH14   AG14   200m   0
|Differential signal data for cell BMLBLVDS18_SSCEH
|MLBP_SIG_N   MLBP_SIG_P
AC2   AC1   200m   NA
|MLBP_DAT_P   MLBP_DAT_N
AA1   AA2   200m   NA
|Differential signal data for cell ILVDS18HY_SSCEH
|MLBP_CLK_N   MLBP_CLK_P
AB2   AB1   200m   NA
|Differential signal data for cell HDMITXPHY
|HDMI1_DATA1X   HDMI1_DATA1Y
AG18   AH18   0.0V   0.0s
|HDMI1_CLOCKX   HDMI1_CLOCKY
AG16   AH16   0.0V   0.0s
|HDMI1_DATA0X   HDMI1_DATA0Y
AG17   AH17   0.0V   0.0s
|HDMI1_DATA2X   HDMI1_DATA2Y
AG19   AH19   0.0V   0.0s
|Differential signal data for cell DDR_DIFFIOPB_H
|DDR1_DQS_ECC   DDR1_DQSN_ECC
V27   V28   200m   0
|DDR2_DQS0   DDR2_DQSN0
G28   G27   200m   0
|DDR1_DQS2   DDR1_DQSN2
AD27   AD28   200m   0
|DDR1_DQS0   DDR1_DQSN0
AH25   AG25   200m   0
|DDR2_DQS3   DDR2_DQSN3
M28   M27   200m   0
|DDR1_DQS3   DDR1_DQSN3
Y28   Y27   200m   0
|DDR2_DQS1   DDR2_DQSN1
H27   H28   200m   0
|DDR1_DQS1   DDR1_DQSN1
AE27   AE28   200m   0
|DDR2_DQS2   DDR2_DQSN2
K27   K28   200m   0
|DDR2_CK   DDR2_NCK
T28   T27   200m   0
|Differential signal data for cell USB2PHYCORE_HMAV10GS80
|USB2_DP   USB2_DM
AE11   AF11   200mV 0ns 0ns 0ns
|USB1_DP   USB1_DM
AD12   AC12   200mV 0ns 0ns 0ns
|Differential signal data for cell GANGARX
|USB_RXP0   USB_RXN0
AE12   AF12   100mV  NA
|PCIE_RXP1   PCIE_RXN1
AH11   AG11   100mV  NA
|PCIE_RXP0   PCIE_RXN0
AH13   AG13   100mV  NA
|SATA1_RXP0   SATA1_RXN0
AG9   AH9   100mV  NA
|Differential signal data for cell SATATX
|SATA1_TXP0   SATA1_TXN0
AH10   AG10   200m   0
|Differential signal data for cell ACSPCIE_RX
|LJCB_CLKP   LJCB_CLKN
AG15   AH15   150m   NA   NA   NA
|Differential signal data for cell DDR_DIFFIOPB_V
|DDR1_CK   DDR1_NCK
AG24   AH24   200m   0
|   Usage I/O#1.8/3.3###BC1833DV40DCPBFBP1811_SSCEV.PAD
|   Base model BC1833DV40DCPBFBP1811_SSCEV
[Model Selector] Selector_1
BC40D_V_10P_!SC1_1P8_M#562 I/O,1.8V,40D CLASS MODE FAST MODE,IND,10 PERCENT%,BC40D_V_10P_!SC1_1P8
BC40D_V_10P_SC1_1P8_M#563 I/O,1.8V,40C CLASS MODE SLOW MODE,IND,10 PERCENT%,BC40D_V_10P_SC1_1P8
BC40D_V_5P_!SC1_1P8_M#564 I/O,1.8V,40D CLASS MODE FAST MODE,IND,5 PERCENT%,BC40D_V_5P_!SC1_1P8
BC40D_V_5P_SC1_1P8_M#565 I/O,1.8V,40C CLASS MODE SLOW MODE,IND,5 PERCENT%,BC40D_V_5P_SC1_1P8
BC40D_V_10P_!SC1_3P3_M#566 I/O,3.3V,40D CLASS MODE FAST MODE,IND,10 PERCENT%,BC40D_V_10P_!SC1_3P3
BC40D_V_10P_SC1_3P3_M#567 I/O,3.3V,40C CLASS MODE SLOW MODE,IND,10 PERCENT%,BC40D_V_10P_SC1_3P3
BC40D_V_5P_!SC1_3P3_M#568 I/O,3.3V,40D CLASS MODE FAST MODE,IND,5 PERCENT%,BC40D_V_5P_!SC1_3P3
BC40D_V_5P_SC1_3P3_M#569 I/O,3.3V,40C CLASS MODE SLOW MODE,IND,5 PERCENT%,BC40D_V_5P_SC1_3P3
|   Usage OUTPUT#1.35/1.5/1.8###DDR_DIFFIOPB_V.PADN
|   Base model DDR_DIFFIOPB_V
[Model Selector] Selector_2
SR011_DRV48_1P8_M#662 I/O,1.8V,SR011_DRV48_1P8
SR010_DRV48_1P8_M#663 I/O,1.8V,SR010_DRV48_1P8
SR101_DRV48_1P8_M#664 I/O,1.8V,SR101_DRV48_1P8
SR100_DRV48_1P8_M#665 I/O,1.8V,SR100_DRV48_1P8
SR110_DRV48_1P8_M#666 I/O,1.8V,SR110_DRV48_1P8
SR111_DRV48_1P8_M#667 I/O,1.8V,SR111_DRV48_1P8
SR001_DRV48_1P8_M#668 I/O,1.8V,SR001_DRV48_1P8
SR000_DRV48_1P8_M#669 I/O,1.8V,SR000_DRV48_1P8
SR011_DRV40_1P8_M#670 I/O,1.8V,SR011_DRV40_1P8
SR010_DRV40_1P8_M#671 I/O,1.8V,SR010_DRV40_1P8
SR101_DRV40_1P8_M#672 I/O,1.8V,SR101_DRV40_1P8
SR100_DRV40_1P8_M#673 I/O,1.8V,SR100_DRV40_1P8
SR110_DRV40_1P8_M#674 I/O,1.8V,SR110_DRV40_1P8
SR111_DRV40_1P8_M#675 I/O,1.8V,SR111_DRV40_1P8
SR001_DRV40_1P8_M#676 I/O,1.8V,SR001_DRV40_1P8
SR000_DRV40_1P8_M#677 I/O,1.8V,SR000_DRV40_1P8
SR011_DRV34_1P8_M#678 I/O,1.8V,SR011_DRV34_1P8
SR010_DRV34_1P8_M#679 I/O,1.8V,SR010_DRV34_1P8
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| Models and submodels in the file (413): USB3_TX_FS_NO_DEEMPHASIS_M#1 (3-state), USB3_TX_FS_3p5_DEEMPHASIS_M#2 (3-state), USB3_TX_HS_NO_DEEMPHASIS_M#3 (3-state), PCIEGEN1_TX_FS_NO_DEEMPHASIS_1p2v_M#4 (3-state), PCIEGEN1_TX_FS_NO_DEEMPHASIS_0p8v_M#5 (3-state), PCIEGEN1_TX_FS_NO_DEEMPHASIS_0p6v_M#6 (3-state), PCIEGEN1_TX_FS_NO_DEEMPHASIS_0p4v_M#7 (3-state), PCIEGEN1_TX_FS_3p5_DEEMPHASIS_1p2v_M#8 (3-state), PCIEGEN1_TX_FS_3p5_DEEMPHASIS_0p8v_M#9 (3-state), PCIEGEN1_TX_FS_3p5_DEEMPHASIS_0p6v_M#10 (3-state), PCIEGEN1_TX_FS_3p5_DEEMPHASIS_0p4v_M#11 (3-state), PCIEGEN1_TX_HS_NO_DEEMPHASIS_0p6v_M#12 (3-state), PCIEGEN1_TX_HS_NO_DEEMPHASIS_0p4v_M#13 (3-state), PCIEGEN1_TX_HS_NO_DEEMPHASIS_0p3v_M#14 (3-state), PCIEGEN1_TX_HS_NO_DEEMPHASIS_0p2v_M#15 (3-state), PCIEGEN2_TX_FS_NO_DEEMPHASIS_1p2v_M#16 (3-state), PCIEGEN2_TX_FS_NO_DEEMPHASIS_0p8v_M#17 (3-state), PCIEGEN2_TX_FS_NO_DEEMPHASIS_0p6v_M#18 (3-state), PCIEGEN2_TX_FS_NO_DEEMPHASIS_0p4v_M#19 (3-state), PCIEGEN2_TX_FS_3p5_DEEMPHASIS_1p2v_M#20 (3-state), PCIEGEN2_TX_FS_3p5_DEEMPHASIS_0p8v_M#21 (3-state), PCIEGEN2_TX_FS_3p5_DEEMPHASIS_0p6v_M#22 (3-state), PCIEGEN2_TX_FS_3p5_DEEMPHASIS_0p4v_M#23 (3-state), PCIEGEN2_TX_FS_6p0_DEEMPHASIS_1p2v_M#24 (3-state), PCIEGEN2_TX_FS_6p0_DEEMPHASIS_0p8v_M#25 (3-state), PCIEGEN2_TX_FS_6p0_DEEMPHASIS_0p6v_M#26 (3-state), PCIEGEN2_TX_FS_6p0_DEEMPHASIS_0p4v_M#27 (3-state), PCIEGEN2_TX_HS_NO_DEEMPHASIS_0p6v_M#28 (3-state), PCIEGEN2_TX_HS_NO_DEEMPHASIS_0p4v_M#29 (3-state), PCIEGEN2_TX_HS_NO_DEEMPHASIS_0p3v_M#30 (3-state), PCIEGEN2_TX_HS_NO_DEEMPHASIS_0p2v_M#31 (3-state), DRIVER_LVL0 (3-state), DRIVER_LVL1 (3-state), DRIVER_LVL2 (3-state), DRIVER_LVL3 (3-state), DRIVER_LVL4 (3-state), DRIVER_LVL5 (3-state), DRIVER_LVL6 (3-state), IQ1833_V_10P_1P8_M#39 (Input), IQ1833_V_5P_1P8_M#40 (Input), IQ1833_V_10P_3P3_M#41 (Input), IQ1833_V_5P_3P3_M#42 (Input), ibis_tmdsp_M#43 (Open_drain), ibis_tmdsm_M#44 (Open_drain), SR011_DRV48_1P8_M#125 (I/O), SR010_DRV48_1P8_M#126 (I/O), SR101_DRV48_1P8_M#127 (I/O), SR100_DRV48_1P8_M#128 (I/O), SR110_DRV48_1P8_M#129 (I/O), SR111_DRV48_1P8_M#130 (I/O), SR001_DRV48_1P8_M#131 (I/O), SR000_DRV48_1P8_M#132 (I/O), SR011_DRV40_1P8_M#133 (I/O), SR010_DRV40_1P8_M#134 (I/O), SR101_DRV40_1P8_M#135 (I/O), SR100_DRV40_1P8_M#136 (I/O), SR110_DRV40_1P8_M#137 (I/O), SR111_DRV40_1P8_M#138 (I/O), SR001_DRV40_1P8_M#139 (I/O), SR000_DRV40_1P8_M#140 (I/O), SR011_DRV34_1P8_M#141 (I/O), SR010_DRV34_1P8_M#142 (I/O), SR101_DRV34_1P8_M#143 (I/O), SR100_DRV34_1P8_M#144 (I/O), SR110_DRV34_1P8_M#145 (I/O), SR111_DRV34_1P8_M#146 (I/O), SR001_DRV34_1P8_M#147 (I/O), SR000_DRV34_1P8_M#148 (I/O), DDR3_ODT_80_1P5_M#149 (Input), DDR3_ODT_60_1P5_M#150 (Input), DDR3_ODT_120_1P5_M#151 (Input), DDR3L_ODT_80_1P35_M#152 (Input), DDR3L_ODT_60_1P35_M#153 (Input), DDR3L_ODT_120_1P35_M#154 (Input), DDR2_ODT_120_1P8_M#155 (Input), DDR2_ODT_80_1P8_M#156 (Input), DDR2_ODT_60_1P8_M#157 (Input), SR011_DRV40_1P5_M#158 (I/O), SR010_DRV40_1P5_M#159 (I/O), SR101_DRV40_1P5_M#160 (I/O)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
